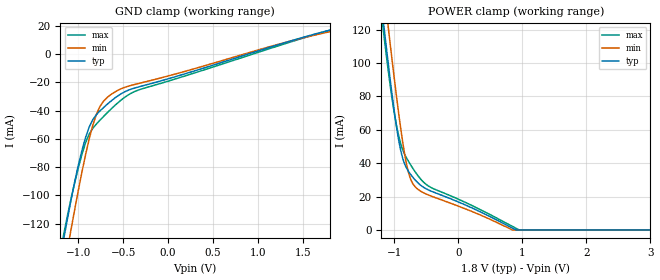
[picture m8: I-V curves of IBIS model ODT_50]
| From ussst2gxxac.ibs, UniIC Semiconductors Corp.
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|   Model ODT_50
[Model]  ODT_50
Model_type Input
Polarity   Non-Inverting
Vinl =   0.70000000V
Vinh =   1.10000000V
C_comp   2.5240pF   2.5060pF   2.5510pF
[Temperature Range]   25.0000   95.0000   0.0
[Voltage Range]   1.8000V   1.7000V   1.9000V
[GND_clamp]
|Voltage   I(typ)   I(min)   I(max)
-1.8V     -372.1mA   -395mA     -366.2mA
-1.16V    -129.6mA   -152mA     -126.4mA
-1.12V    -115.9mA   -137.6mA   -113.8mA
-1.08V    -102.6mA   -123.5mA   -101.9mA
-960mV    -68.15mA   -83.38mA   -70.89mA
-880mV    -51.76mA   -60.19mA   -56.67mA
-840mV    -46.5mA    -50.56mA   -52.63mA
-760mV    -40.33mA   -37.15mA   -46.88mA
-600mV    -31.48mA   -27.15mA   -36.81mA
-440mV    -25.53mA   -22.73mA   -28.79mA
-320mV    -23.16mA   -20.75mA   -25.28mA
1.8V      16.81mA    15.75mA    16.73mA
[POWER_clamp]
|Voltage   I(typ)   I(min)   I(max)
-1.8V     350.9mA    373.4mA    344.4mA
-1.18V    129mA      151.5mA    123.5mA
-1.14V    115.5mA    137.8mA    110.5mA
-1.08V    95.97mA    117.6mA    91.95mA
-1V       71.74mA    91.61mA    70.67mA
-920mV    51.99mA    67.32mA    55.06mA
-860mV    42.18mA    51.18mA    47.4mA
-800mV    36.62mA    38.31mA    42.71mA
-720mV    32.15mA    28.55mA    37.64mA
-580mV    26.6mA     23.08mA    30.23mA
903.9mV   0A         NA         NA
3.6V      0A         0A         0A
